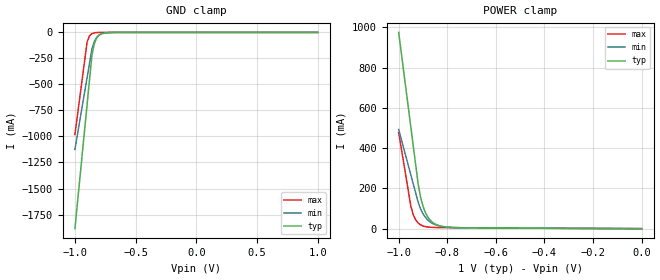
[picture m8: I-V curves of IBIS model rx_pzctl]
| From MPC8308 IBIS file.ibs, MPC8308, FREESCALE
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[Model]   rx_pzctl
Model_type Input
Vinh=0.8
Vinl=0.2
C_comp   777.9fF   774fF   777.9fF
[Model Spec]
[Temperature Range] 65   125   -40
[Voltage Range]   1   0.9   1.1
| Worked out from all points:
|   GND clamp passes 1 mA (typ) near -0.71 V on its own axis
|   POWER clamp passes 1 mA (typ) near -0.20 V on its own axis
[GND Clamp]
-1V       -1.886A    -1.124A    -981.3mA
-900mV    -696.3mA   -435.6mA   -93.85mA
-880mV    -458.4mA   -297.9mA   -32.63mA
-860mV    -220.6mA   -160.2mA   -11.39mA
-840mV    -106.3mA   -86.22mA   -4.002mA
-820mV    -51.36mA   -46.49mA   -1.413mA
-800mV    -24.85mA   -25.08mA   -481.4uA
-760mV    -5.87mA    -7.326mA   -70.31uA
-680mV    -314.2uA   -587.5uA   0A
1V        0A         0A         0A
[POWER Clamp]
-1V       974.6mA    492.6mA    477.8mA
-950mV    505.1mA    267.3mA    112.4mA
-940mV    411.2mA    222.2mA    69.07mA
-930mV    317.3mA    177.1mA    43.37mA
-920mV    223.3mA    132.1mA    28.09mA
-910mV    157.7mA    98.79mA    18.98mA
-900mV    111.9mA    74.22mA    13.53mA
-880mV    57.36mA    42.63mA    8.272mA
-860mV    30.62mA    25.33mA    6.309mA
-820mV    10.9mA     10.56mA    5.149mA
-760mV    5.039mA    5mA        4.598mA
0V        24.64nA    6.313nA    131.3nA
